(* Logix 5000 AddOnInstructionDefinition export Banner_RSio_ISD_Device_Type_in_Chain_v1; software revision 33.00 *)

TYPE Banner_RSio_ISD_Device_Types_v1 :
STRUCT
   Chain : SINT;   // Enter Chain that will be accessed.
   Access_Chain : SINT;
   Devices_in_Chain : SINT[32];
END_STRUCT
END_TYPE

ADD_ON_INSTRUCTION Banner_RSio_ISD_Device_Type_in_Chain_v1   (* revision 1.0 *)
VAR_IN_OUT
   ChainDevices : Banner_RSio_ISD_Device_Types_v1; {required}
   MSG : MESSAGE; {required}
   Activate : BOOL; {required}
END_VAR
VAR_OUTPUT
   Busy : BOOL; {visible}
   Done : BOOL; {visible}
   Error : BOOL; {visible}
END_VAR
VAR
   Timer : TIMER := (PRE := 5000); {access None}
   Control : DINT; {access None}
END_VAR

ROUTINE Logic   (* ladder *)
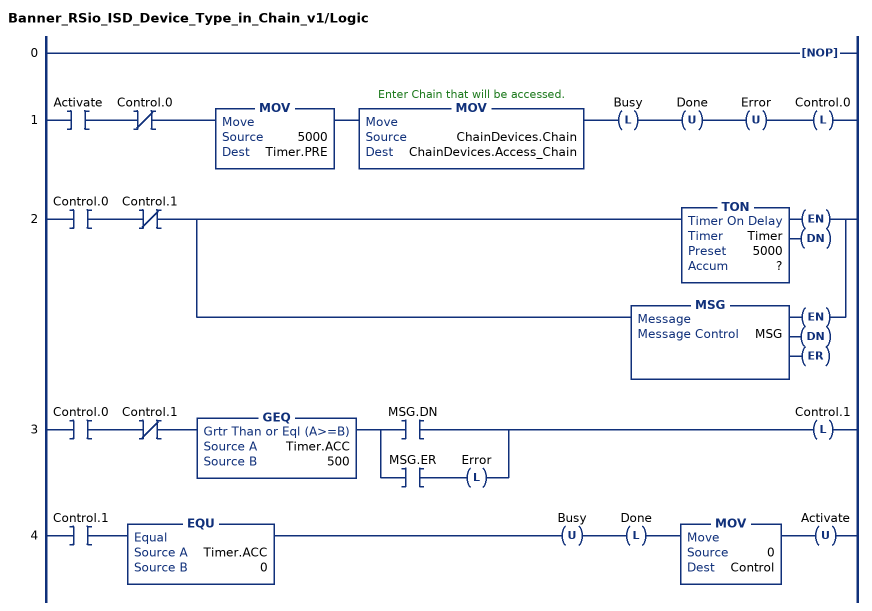
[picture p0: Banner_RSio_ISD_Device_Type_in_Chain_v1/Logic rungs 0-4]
   0: NOP();
   1: XIC(Activate)XIO(Control.0)MOV(5000,Timer.PRE)MOV(ChainDevices.Chain,ChainDevices.Access_Chain)OTL(Busy)OTU(Done)OTU(Error)OTL(Control.0);
   2: XIC(Control.0)XIO(Control.1)[TON(Timer,?,?) ,MSG(MSG) ];
   3: XIC(Control.0)XIO(Control.1)GEQ(Timer.ACC,500)[XIC(MSG.DN) ,XIC(MSG.ER) OTL(Error) ]OTL(Control.1);
   4: XIC(Control.1)EQU(Timer.ACC,0)OTU(Busy)OTL(Done)MOV(0,Control)OTU(Activate);
END_ROUTINE
END_ADD_ON_INSTRUCTION
